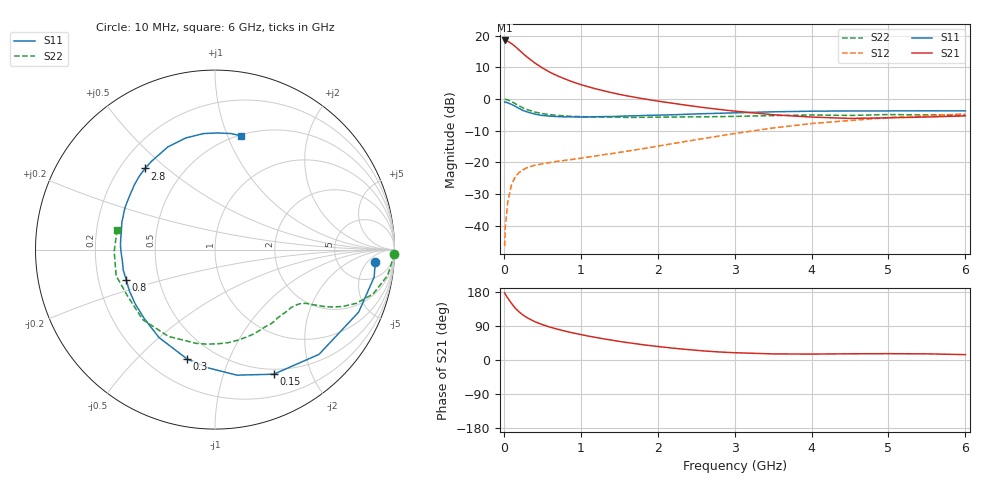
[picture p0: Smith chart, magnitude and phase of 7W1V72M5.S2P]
! Infineon Technologies  Discrete & RF Semiconductors
! BFS17W
! Si NPN RF Bipolar Junction Transistor in SOT323
! VCE = 1.75 V  IC = 2.5 mA
! Common Emitter S-Parameters:  August  1999
# GHz  S  MA  R  50
!  f  S11  S21  S12  S22
! GHz  MAG  ANG  MAG  ANG  MAG  ANG  MAG  ANG
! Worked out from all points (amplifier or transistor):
!   36 points, 10 MHz to 6 GHz, reference 50 ohm
!   highest |S21| = 18.5 dB at 10 MHz (marker M1)
!   |S21| within 3 dB of that: start of sweep to 198.6 MHz
!   unconditionally stable (mu >= 1): 732.1 MHz to end of sweep
!   at 250 MHz: K = 0.42, MSG = 18.3 dB, |S12| = -22.3 dB
!   at 1.4 GHz: K = 1.34, MAG = 6.1 dB, |S12| = -17.2 dB
!   at 6 GHz: K = 1.11, MAG = -2.3 dB, |S12| = -4.7 dB
!   S11 on the Smith chart (normalised r, x): 10 MHz: 12, -9; 150 MHz: 0.44, -1.48; 300 MHz: 0.35, -0.71; 800 MHz: 0.32, -0.15; 2.8 GHz: 0.30, +0.42; 6 GHz: 0.51, +1.12
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0.01  0.8957 -4.6  8.382 177.4  0.0048 86.5  0.9972 -1.3
0.02  0.8999 -9.8  8.356 173.5  0.0097 86.8  0.9908 -3.5
0.05  0.8729 -23.5  8.156 163.6  0.0235 78.1  0.9718 -8.6
0.1  0.8225 -45.2  7.485 149.2  0.0448 66.4  0.9149 -15.7
0.15  0.7674 -64.8  6.7 136.4  0.0599 57.2  0.8423 -20.8
0.2  0.7101 -80.1  5.913 126.6  0.0699 51.5  0.7792 -24.0
0.25  0.6602 -93.3  5.202 118.5  0.0768 46.4  0.7243 -26.2
0.3  0.6285 -104.4  4.613 111.9  0.0827 43.9  0.6839 -27.6
0.4  0.5809 -122.4  3.721 101.3  0.0903 40.1  0.6248 -29.4
0.5  0.5507 -135.6  3.1 93.4  0.0951 39.2  0.5904 -30.5
0.6  0.5378 -145.8  2.639 86.7  0.0998 39.0  0.5673 -31.9
0.8  0.5227 -161.4  2.061 76.0  0.1081 41.1  0.5404 -35.7
0.9  0.5238 -167.4  1.853 71.4  0.1122 42.2  0.532 -37.6
1.1  0.5228 -177.8  1.557 63.0  0.1223 45.1  0.5236 -42.4
1.3  0.5289 173.6  1.347 55.7  0.1332 47.8  0.5163 -48.0
1.6  0.5416 163.1  1.123 46.1  0.1507 51.6  0.5132 -56.5
2.2  0.5651 146.2  0.856 31.2  0.199 57.2  0.5204 -75.3
2.8  0.5968 130.7  0.686 21.2  0.2614 57.9  0.5286 -95.1
3.5  0.6296 114.6  0.566 16.1  0.3499 54.1  0.5488 -118.2
4.5  0.6497 95.6  0.495 16.4  0.4587 42.6  0.5513 -151.6
5.5  0.6527 82.3  0.521 16.2  0.5479 30.8  0.5618 -179.1
6  0.6505 77.1  0.543 14.2  0.5827 25.2  0.5557 168.8
